(* Logix 5000 AddOnInstructionDefinition export Banner_WLS_Param_v4; software revision 33.00; part 3 of 3 *)
(* tags used below, declared in another part *)
   WLS : Banner_WLS_v4;
   Port_Data : Banner_IOL_Port_v4;
   Port : INT;   // Port Number that device is plugged into.
   Type : SINT;   // 0 = WLS27, 1 = WLS15, 2 = WLF
   Local_Control : DINT;
   Command_Being_Processed : BOOL;
   Update_Archive : BOOL;
   Index_Write_Inprocess : DINT;
   Inprocess_Index : DINT;
   SW_Index : DINT;
   LTW_Index : DINT;
   GW_Index : DINT;
(* Banner_WLS_Param_v4, continued *)

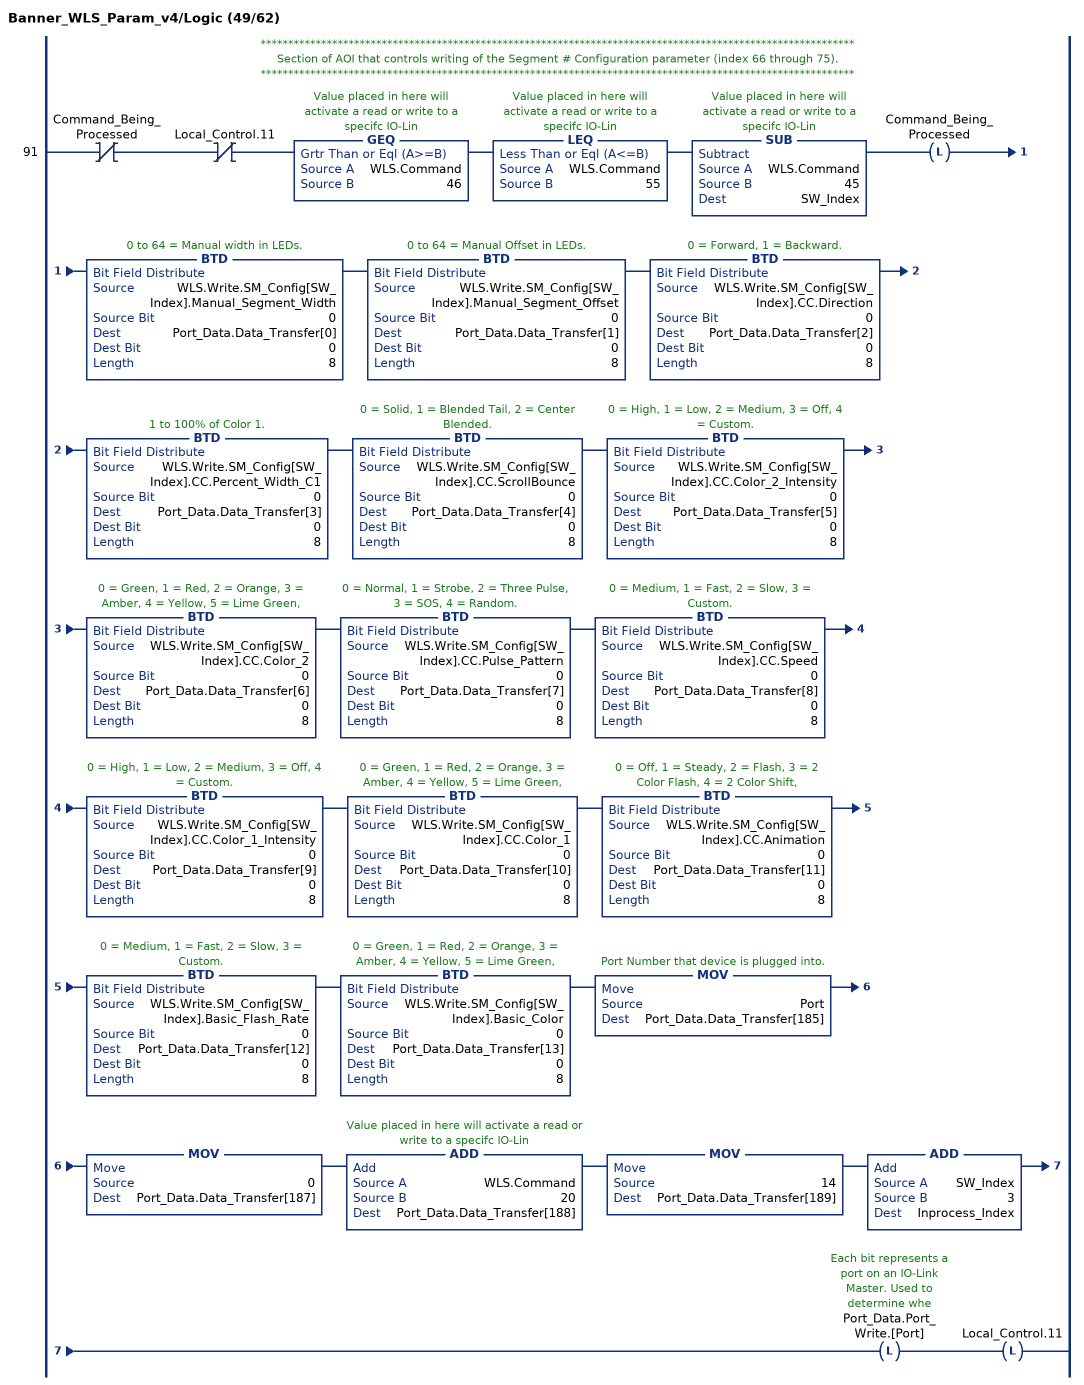
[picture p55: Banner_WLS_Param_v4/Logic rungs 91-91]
   // ************************************************************************************************************
   // Section of AOI that controls writing of the Segment # Configuration parameter (index 66 through 75).
   // ************************************************************************************************************
   91: XIO(Command_Being_Processed)XIO(Local_Control.11)GEQ(WLS.Command,46)LEQ(WLS.Command,55)SUB(WLS.Command,45,SW_Index)OTL(Command_Being_Processed)BTD(WLS.Write.SM_Config[SW_Index].Manual_Segment_Width,0,Port_Data.Data_Transfer[0],0,8)BTD(WLS.Write.SM_Config[SW_Index].Manual_Segment_Offset,0,Port_Data.Data_Transfer[1],0,8)BTD(WLS.Write.SM_Config[SW_Index].CC.Direction,0,Port_Data.Data_Transfer[2],0,8)BTD(WLS.Write.SM_Config[SW_Index].CC.Percent_Width_C1,0,Port_Data.Data_Transfer[3],0,8)BTD(WLS.Write.SM_Config[SW_Index].CC.ScrollBounce,0,Port_Data.Data_Transfer[4],0,8)BTD(WLS.Write.SM_Config[SW_Index].CC.Color_2_Intensity,0,Port_Data.Data_Transfer[5],0,8)BTD(WLS.Write.SM_Config[SW_Index].CC.Color_2,0,Port_Data.Data_Transfer[6],0,8)BTD(WLS.Write.SM_Config[SW_Index].CC.Pulse_Pattern,0,Port_Data.Data_Transfer[7],0,8)BTD(WLS.Write.SM_Config[SW_Index].CC.Speed,0,Port_Data.Data_Transfer[8],0,8)BTD(WLS.Write.SM_Config[SW_Index].CC.Color_1_Intensity,0,Port_Data.Data_Transfer[9],0,8)BTD(WLS.Write.SM_Config[SW_Index].CC.Color_1,0,Port_Data.Data_Transfer[10],0,8)BTD(WLS.Write.SM_Config[SW_Index].CC.Animation,0,Port_Data.Data_Transfer[11],0,8)BTD(WLS.Write.SM_Config[SW_Index].Basic_Flash_Rate,0,Port_Data.Data_Transfer[12],0,8)BTD(WLS.Write.SM_Config[SW_Index].Basic_Color,0,Port_Data.Data_Transfer[13],0,8)MOV(Port,Port_Data.Data_Transfer[185])MOV(0,Port_Data.Data_Transfer[187])ADD(WLS.Command,20,Port_Data.Data_Transfer[188])MOV(14,Port_Data.Data_Transfer[189])ADD(SW_Index,3,Inprocess_Index)OTL(Port_Data.Port_Write.[Port])OTL(Local_Control.11);
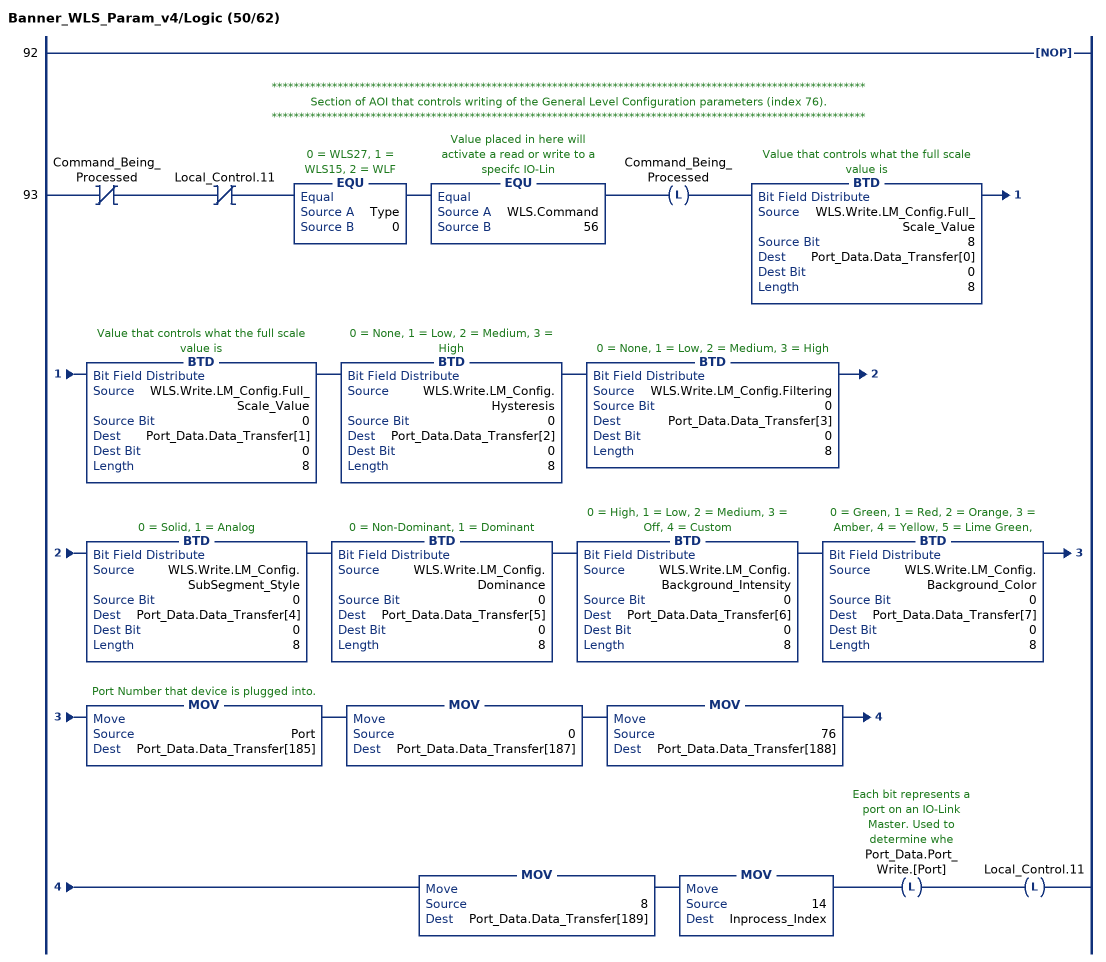
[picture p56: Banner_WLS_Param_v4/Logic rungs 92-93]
   92: NOP();
   // ************************************************************************************************************
   // Section of AOI that controls writing of the General Level Configuration parameters (index 76).
   // ************************************************************************************************************
   93: XIO(Command_Being_Processed)XIO(Local_Control.11)EQU(Type,0)EQU(WLS.Command,56)OTL(Command_Being_Processed)BTD(WLS.Write.LM_Config.Full_Scale_Value,8,Port_Data.Data_Transfer[0],0,8)BTD(WLS.Write.LM_Config.Full_Scale_Value,0,Port_Data.Data_Transfer[1],0,8)BTD(WLS.Write.LM_Config.Hysteresis,0,Port_Data.Data_Transfer[2],0,8)BTD(WLS.Write.LM_Config.Filtering,0,Port_Data.Data_Transfer[3],0,8)BTD(WLS.Write.LM_Config.SubSegment_Style,0,Port_Data.Data_Transfer[4],0,8)BTD(WLS.Write.LM_Config.Dominance,0,Port_Data.Data_Transfer[5],0,8)BTD(WLS.Write.LM_Config.Background_Intensity,0,Port_Data.Data_Transfer[6],0,8)BTD(WLS.Write.LM_Config.Background_Color,0,Port_Data.Data_Transfer[7],0,8)MOV(Port,Port_Data.Data_Transfer[185])MOV(0,Port_Data.Data_Transfer[187])MOV(76,Port_Data.Data_Transfer[188])MOV(8,Port_Data.Data_Transfer[189])MOV(14,Inprocess_Index)OTL(Port_Data.Port_Write.[Port])OTL(Local_Control.11);
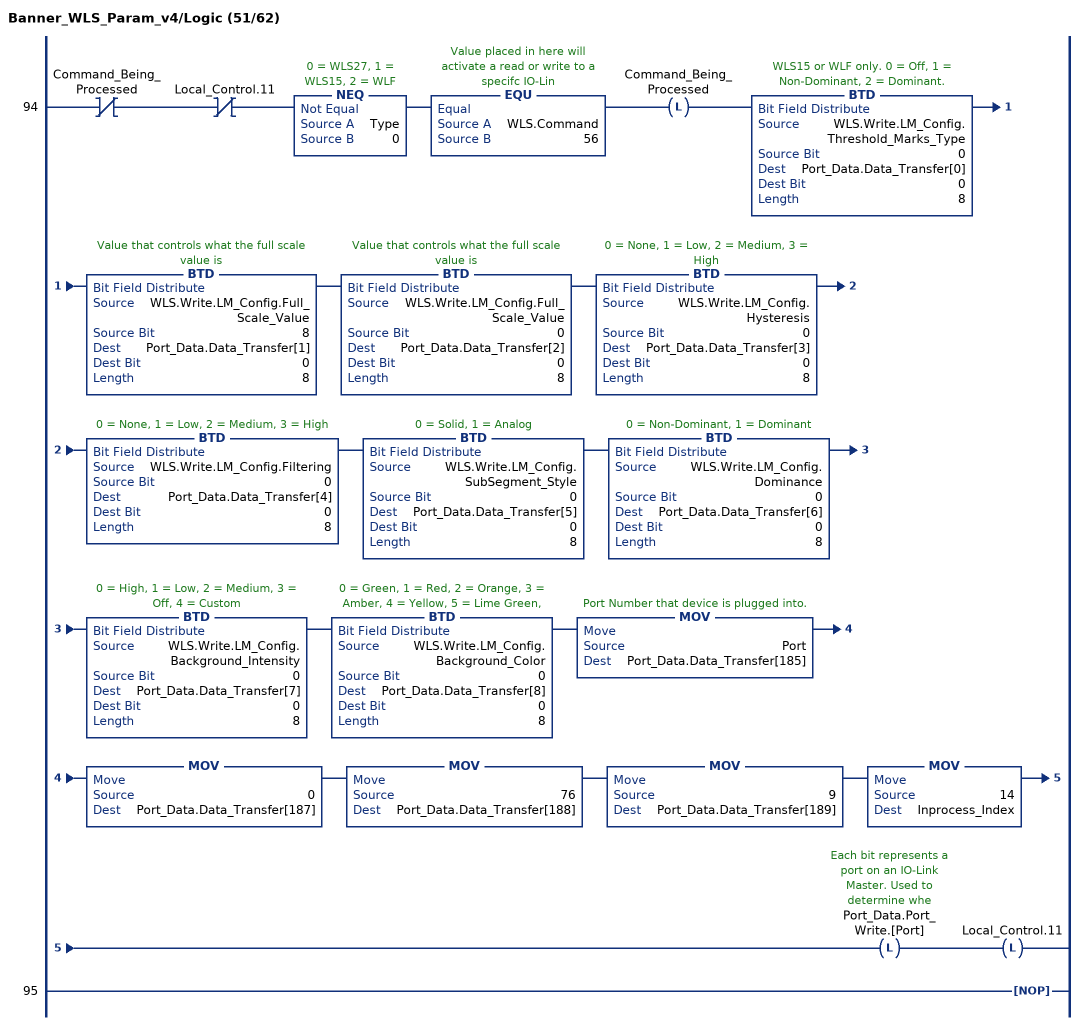
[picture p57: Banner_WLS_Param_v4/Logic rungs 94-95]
   94: XIO(Command_Being_Processed)XIO(Local_Control.11)NEQ(Type,0)EQU(WLS.Command,56)OTL(Command_Being_Processed)BTD(WLS.Write.LM_Config.Threshold_Marks_Type,0,Port_Data.Data_Transfer[0],0,8)BTD(WLS.Write.LM_Config.Full_Scale_Value,8,Port_Data.Data_Transfer[1],0,8)BTD(WLS.Write.LM_Config.Full_Scale_Value,0,Port_Data.Data_Transfer[2],0,8)BTD(WLS.Write.LM_Config.Hysteresis,0,Port_Data.Data_Transfer[3],0,8)BTD(WLS.Write.LM_Config.Filtering,0,Port_Data.Data_Transfer[4],0,8)BTD(WLS.Write.LM_Config.SubSegment_Style,0,Port_Data.Data_Transfer[5],0,8)BTD(WLS.Write.LM_Config.Dominance,0,Port_Data.Data_Transfer[6],0,8)BTD(WLS.Write.LM_Config.Background_Intensity,0,Port_Data.Data_Transfer[7],0,8)BTD(WLS.Write.LM_Config.Background_Color,0,Port_Data.Data_Transfer[8],0,8)MOV(Port,Port_Data.Data_Transfer[185])MOV(0,Port_Data.Data_Transfer[187])MOV(76,Port_Data.Data_Transfer[188])MOV(9,Port_Data.Data_Transfer[189])MOV(14,Inprocess_Index)OTL(Port_Data.Port_Write.[Port])OTL(Local_Control.11);
   95: NOP();
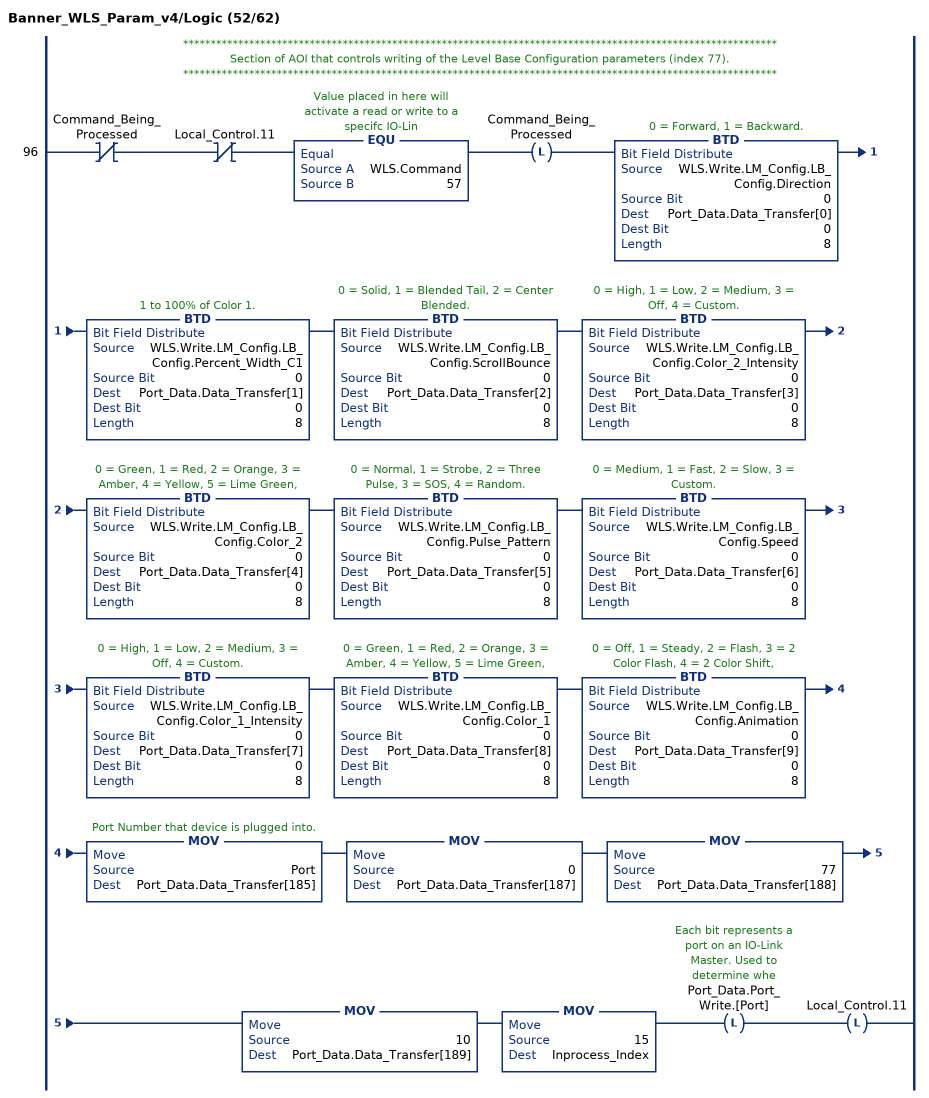
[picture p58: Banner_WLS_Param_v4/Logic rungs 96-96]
   // ************************************************************************************************************
   // Section of AOI that controls writing of the Level Base Configuration parameters (index 77).
   // ************************************************************************************************************
   96: XIO(Command_Being_Processed)XIO(Local_Control.11)EQU(WLS.Command,57)OTL(Command_Being_Processed)BTD(WLS.Write.LM_Config.LB_Config.Direction,0,Port_Data.Data_Transfer[0],0,8)BTD(WLS.Write.LM_Config.LB_Config.Percent_Width_C1,0,Port_Data.Data_Transfer[1],0,8)BTD(WLS.Write.LM_Config.LB_Config.ScrollBounce,0,Port_Data.Data_Transfer[2],0,8)BTD(WLS.Write.LM_Config.LB_Config.Color_2_Intensity,0,Port_Data.Data_Transfer[3],0,8)BTD(WLS.Write.LM_Config.LB_Config.Color_2,0,Port_Data.Data_Transfer[4],0,8)BTD(WLS.Write.LM_Config.LB_Config.Pulse_Pattern,0,Port_Data.Data_Transfer[5],0,8)BTD(WLS.Write.LM_Config.LB_Config.Speed,0,Port_Data.Data_Transfer[6],0,8)BTD(WLS.Write.LM_Config.LB_Config.Color_1_Intensity,0,Port_Data.Data_Transfer[7],0,8)BTD(WLS.Write.LM_Config.LB_Config.Color_1,0,Port_Data.Data_Transfer[8],0,8)BTD(WLS.Write.LM_Config.LB_Config.Animation,0,Port_Data.Data_Transfer[9],0,8)MOV(Port,Port_Data.Data_Transfer[185])MOV(0,Port_Data.Data_Transfer[187])MOV(77,Port_Data.Data_Transfer[188])MOV(10,Port_Data.Data_Transfer[189])MOV(15,Inprocess_Index)OTL(Port_Data.Port_Write.[Port])OTL(Local_Control.11);
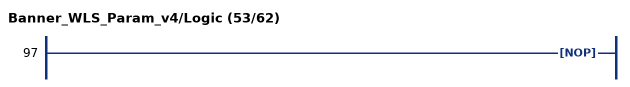
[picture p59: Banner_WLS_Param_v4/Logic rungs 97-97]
   97: NOP();
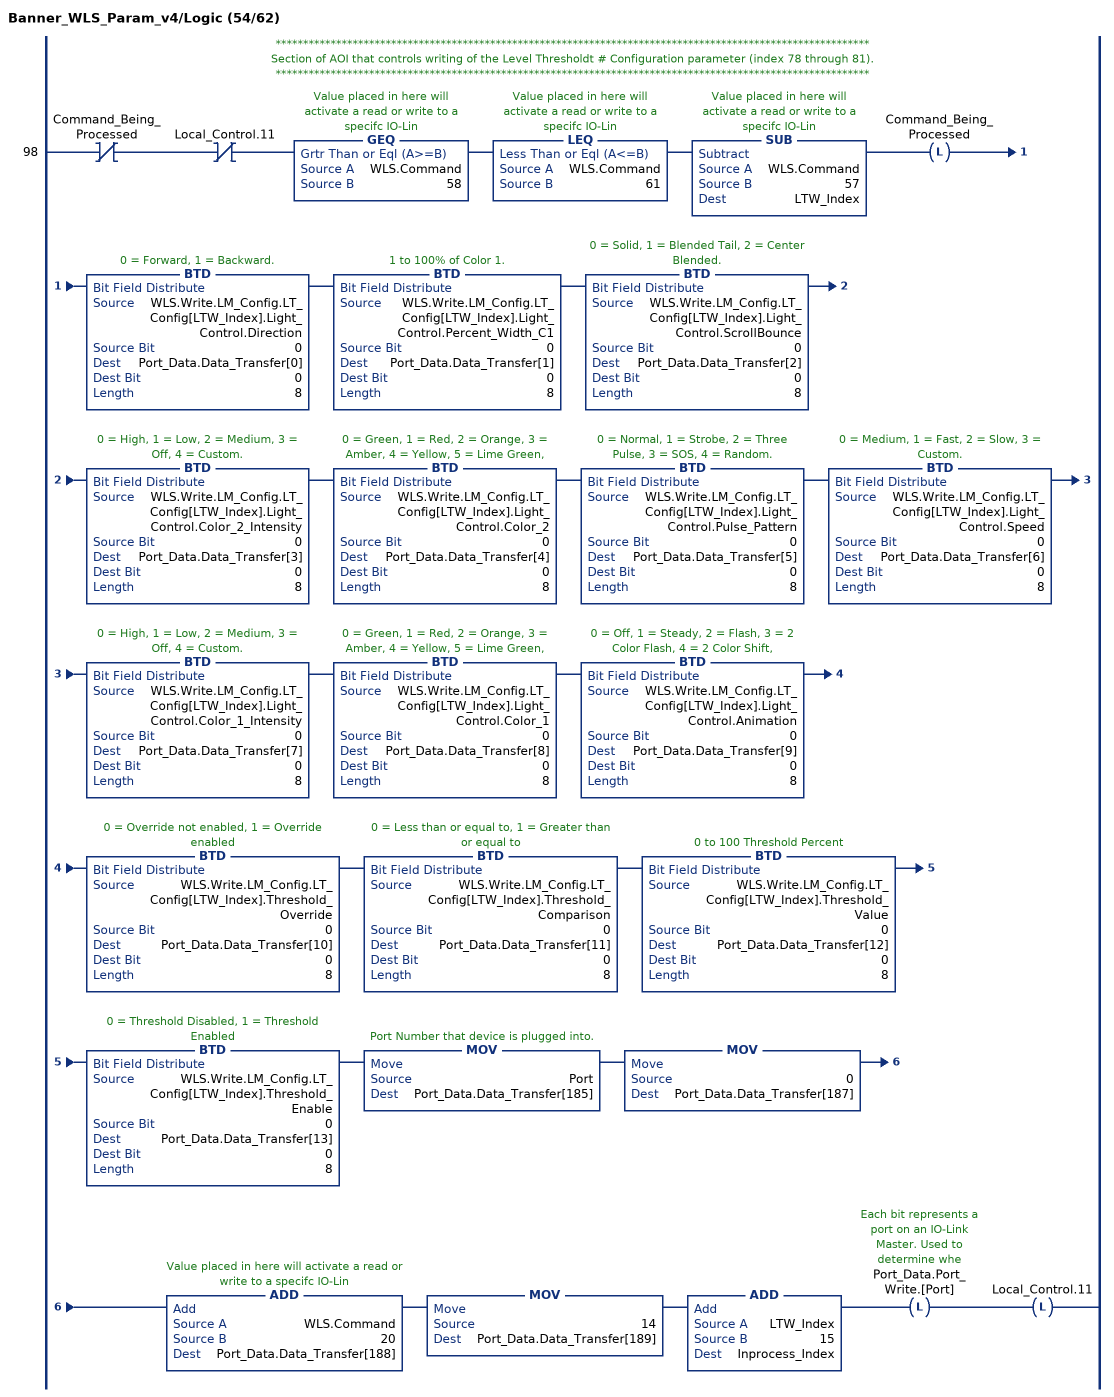
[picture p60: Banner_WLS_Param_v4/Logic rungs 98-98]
   // ************************************************************************************************************
   // Section of AOI that controls writing of the Level Thresholdt # Configuration parameter (index 78 through 81).
   // ************************************************************************************************************
   98: XIO(Command_Being_Processed)XIO(Local_Control.11)GEQ(WLS.Command,58)LEQ(WLS.Command,61)SUB(WLS.Command,57,LTW_Index)OTL(Command_Being_Processed)BTD(WLS.Write.LM_Config.LT_Config[LTW_Index].Light_Control.Direction,0,Port_Data.Data_Transfer[0],0,8)BTD(WLS.Write.LM_Config.LT_Config[LTW_Index].Light_Control.Percent_Width_C1,0,Port_Data.Data_Transfer[1],0,8)BTD(WLS.Write.LM_Config.LT_Config[LTW_Index].Light_Control.ScrollBounce,0,Port_Data.Data_Transfer[2],0,8)BTD(WLS.Write.LM_Config.LT_Config[LTW_Index].Light_Control.Color_2_Intensity,0,Port_Data.Data_Transfer[3],0,8)BTD(WLS.Write.LM_Config.LT_Config[LTW_Index].Light_Control.Color_2,0,Port_Data.Data_Transfer[4],0,8)BTD(WLS.Write.LM_Config.LT_Config[LTW_Index].Light_Control.Pulse_Pattern,0,Port_Data.Data_Transfer[5],0,8)BTD(WLS.Write.LM_Config.LT_Config[LTW_Index].Light_Control.Speed,0,Port_Data.Data_Transfer[6],0,8)BTD(WLS.Write.LM_Config.LT_Config[LTW_Index].Light_Control.Color_1_Intensity,0,Port_Data.Data_Transfer[7],0,8)BTD(WLS.Write.LM_Config.LT_Config[LTW_Index].Light_Control.Color_1,0,Port_Data.Data_Transfer[8],0,8)BTD(WLS.Write.LM_Config.LT_Config[LTW_Index].Light_Control.Animation,0,Port_Data.Data_Transfer[9],0,8)BTD(WLS.Write.LM_Config.LT_Config[LTW_Index].Threshold_Override,0,Port_Data.Data_Transfer[10],0,8)BTD(WLS.Write.LM_Config.LT_Config[LTW_Index].Threshold_Comparison,0,Port_Data.Data_Transfer[11],0,8)BTD(WLS.Write.LM_Config.LT_Config[LTW_Index].Threshold_Value,0,Port_Data.Data_Transfer[12],0,8)BTD(WLS.Write.LM_Config.LT_Config[LTW_Index].Threshold_Enable,0,Port_Data.Data_Transfer[13],0,8)MOV(Port,Port_Data.Data_Transfer[185])MOV(0,Port_Data.Data_Transfer[187])ADD(WLS.Command,20,Port_Data.Data_Transfer[188])MOV(14,Port_Data.Data_Transfer[189])ADD(LTW_Index,15,Inprocess_Index)OTL(Port_Data.Port_Write.[Port])OTL(Local_Control.11);
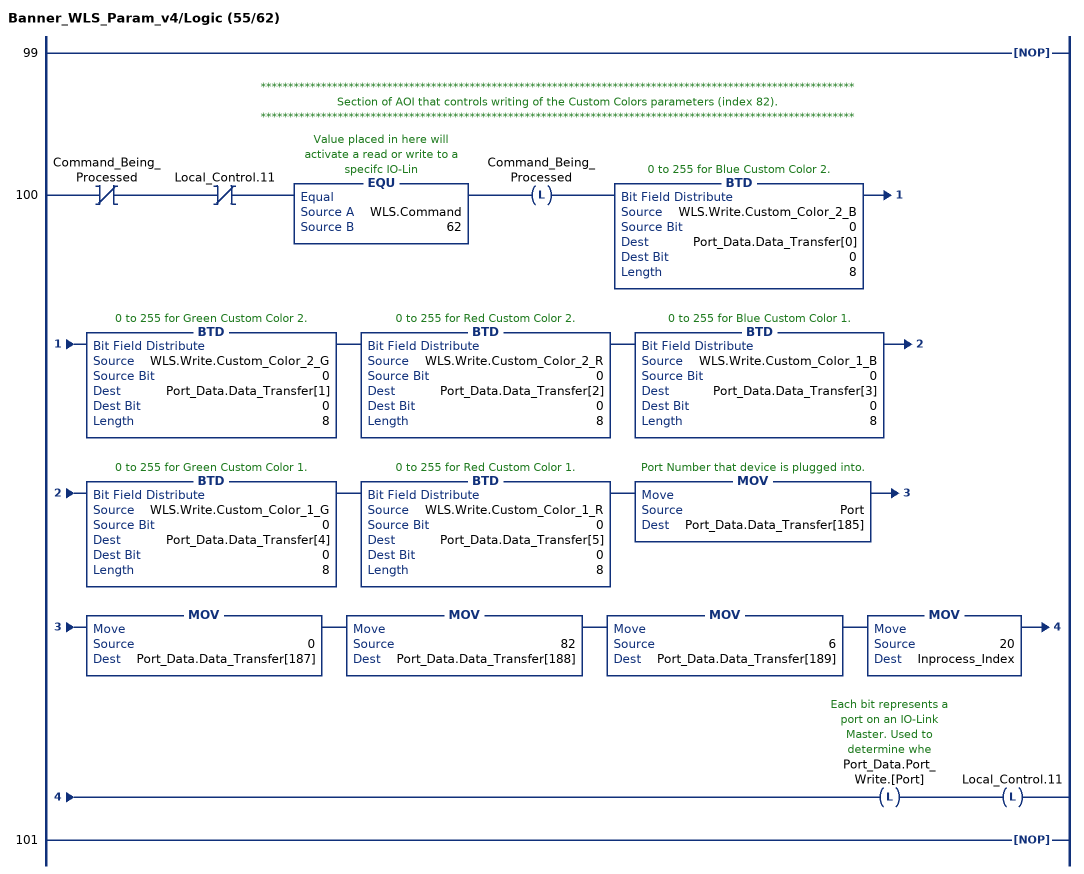
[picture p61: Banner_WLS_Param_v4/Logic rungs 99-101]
   99: NOP();
   // ************************************************************************************************************
   // Section of AOI that controls writing of the Custom Colors parameters (index 82).
   // ************************************************************************************************************
   100: XIO(Command_Being_Processed)XIO(Local_Control.11)EQU(WLS.Command,62)OTL(Command_Being_Processed)BTD(WLS.Write.Custom_Color_2_B,0,Port_Data.Data_Transfer[0],0,8)BTD(WLS.Write.Custom_Color_2_G,0,Port_Data.Data_Transfer[1],0,8)BTD(WLS.Write.Custom_Color_2_R,0,Port_Data.Data_Transfer[2],0,8)BTD(WLS.Write.Custom_Color_1_B,0,Port_Data.Data_Transfer[3],0,8)BTD(WLS.Write.Custom_Color_1_G,0,Port_Data.Data_Transfer[4],0,8)BTD(WLS.Write.Custom_Color_1_R,0,Port_Data.Data_Transfer[5],0,8)MOV(Port,Port_Data.Data_Transfer[185])MOV(0,Port_Data.Data_Transfer[187])MOV(82,Port_Data.Data_Transfer[188])MOV(6,Port_Data.Data_Transfer[189])MOV(20,Inprocess_Index)OTL(Port_Data.Port_Write.[Port])OTL(Local_Control.11);
   101: NOP();
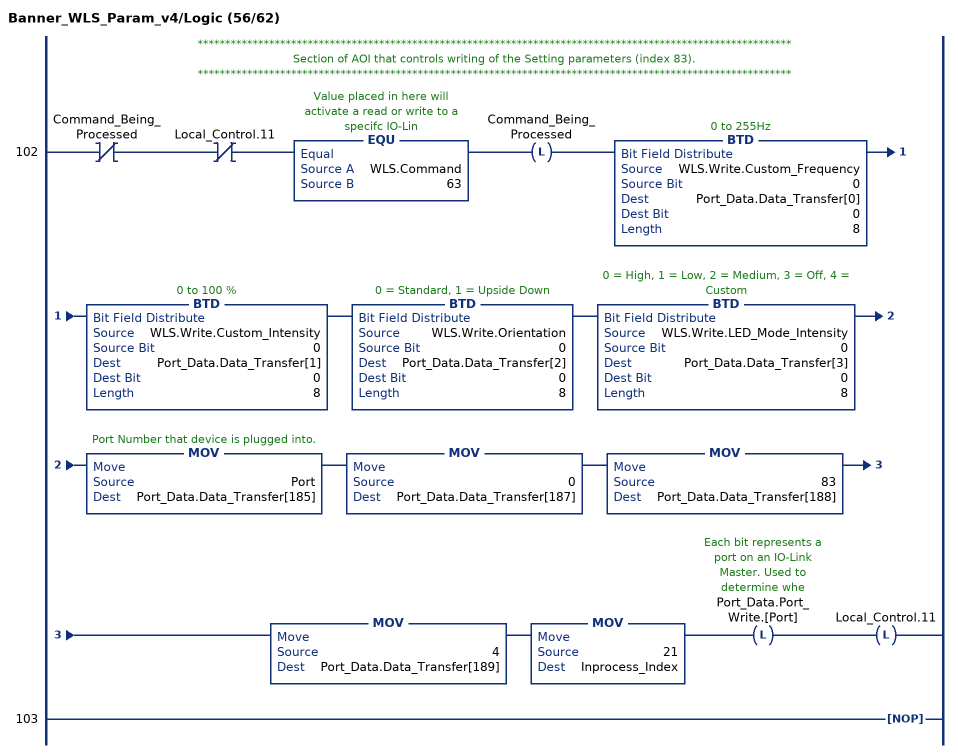
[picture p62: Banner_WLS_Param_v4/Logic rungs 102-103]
   // ************************************************************************************************************
   // Section of AOI that controls writing of the Setting parameters (index 83).
   // ************************************************************************************************************
   102: XIO(Command_Being_Processed)XIO(Local_Control.11)EQU(WLS.Command,63)OTL(Command_Being_Processed)BTD(WLS.Write.Custom_Frequency,0,Port_Data.Data_Transfer[0],0,8)BTD(WLS.Write.Custom_Intensity,0,Port_Data.Data_Transfer[1],0,8)BTD(WLS.Write.Orientation,0,Port_Data.Data_Transfer[2],0,8)BTD(WLS.Write.LED_Mode_Intensity,0,Port_Data.Data_Transfer[3],0,8)MOV(Port,Port_Data.Data_Transfer[185])MOV(0,Port_Data.Data_Transfer[187])MOV(83,Port_Data.Data_Transfer[188])MOV(4,Port_Data.Data_Transfer[189])MOV(21,Inprocess_Index)OTL(Port_Data.Port_Write.[Port])OTL(Local_Control.11);
   103: NOP();
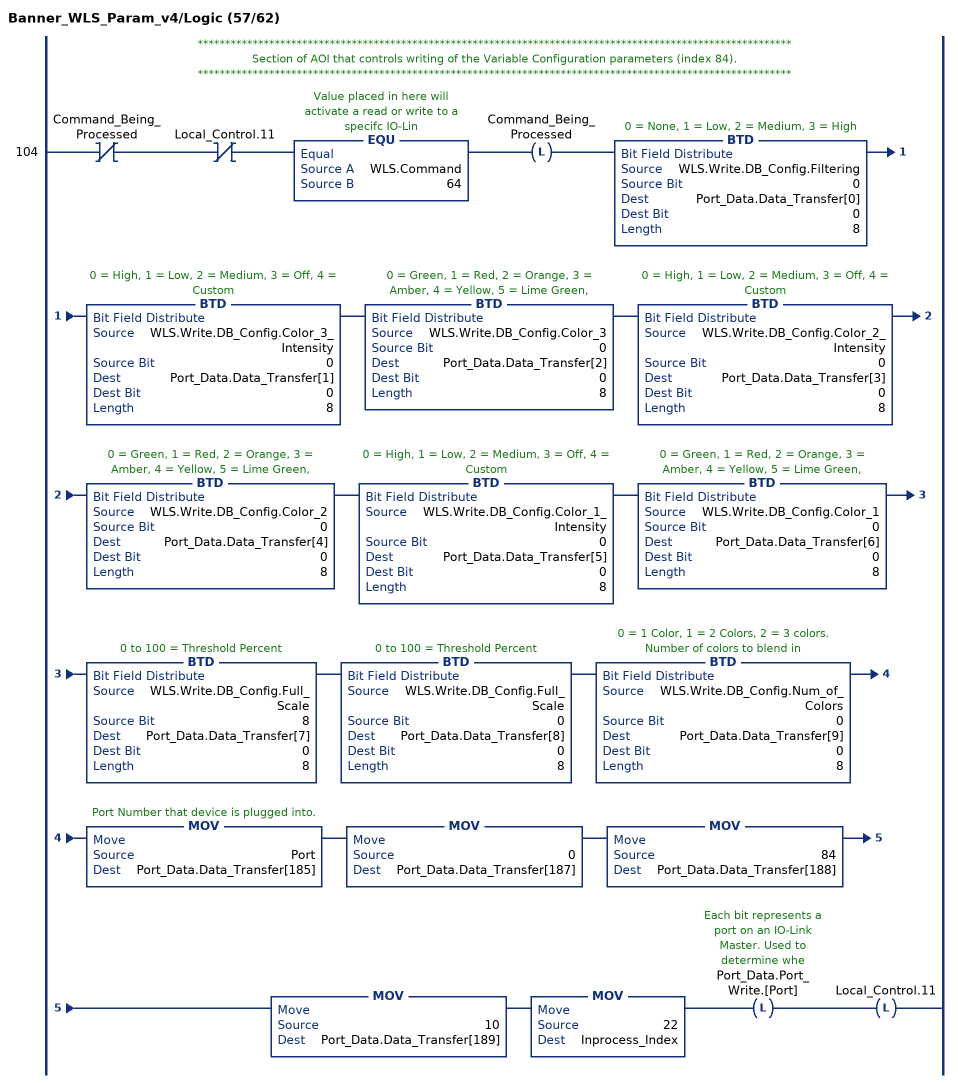
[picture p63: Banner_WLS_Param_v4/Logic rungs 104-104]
   // ************************************************************************************************************
   // Section of AOI that controls writing of the Variable Configuration parameters (index 84).
   // ************************************************************************************************************
   104: XIO(Command_Being_Processed)XIO(Local_Control.11)EQU(WLS.Command,64)OTL(Command_Being_Processed)BTD(WLS.Write.DB_Config.Filtering,0,Port_Data.Data_Transfer[0],0,8)BTD(WLS.Write.DB_Config.Color_3_Intensity,0,Port_Data.Data_Transfer[1],0,8)BTD(WLS.Write.DB_Config.Color_3,0,Port_Data.Data_Transfer[2],0,8)BTD(WLS.Write.DB_Config.Color_2_Intensity,0,Port_Data.Data_Transfer[3],0,8)BTD(WLS.Write.DB_Config.Color_2,0,Port_Data.Data_Transfer[4],0,8)BTD(WLS.Write.DB_Config.Color_1_Intensity,0,Port_Data.Data_Transfer[5],0,8)BTD(WLS.Write.DB_Config.Color_1,0,Port_Data.Data_Transfer[6],0,8)BTD(WLS.Write.DB_Config.Full_Scale,8,Port_Data.Data_Transfer[7],0,8)BTD(WLS.Write.DB_Config.Full_Scale,0,Port_Data.Data_Transfer[8],0,8)BTD(WLS.Write.DB_Config.Num_of_Colors,0,Port_Data.Data_Transfer[9],0,8)MOV(Port,Port_Data.Data_Transfer[185])MOV(0,Port_Data.Data_Transfer[187])MOV(84,Port_Data.Data_Transfer[188])MOV(10,Port_Data.Data_Transfer[189])MOV(22,Inprocess_Index)OTL(Port_Data.Port_Write.[Port])OTL(Local_Control.11);
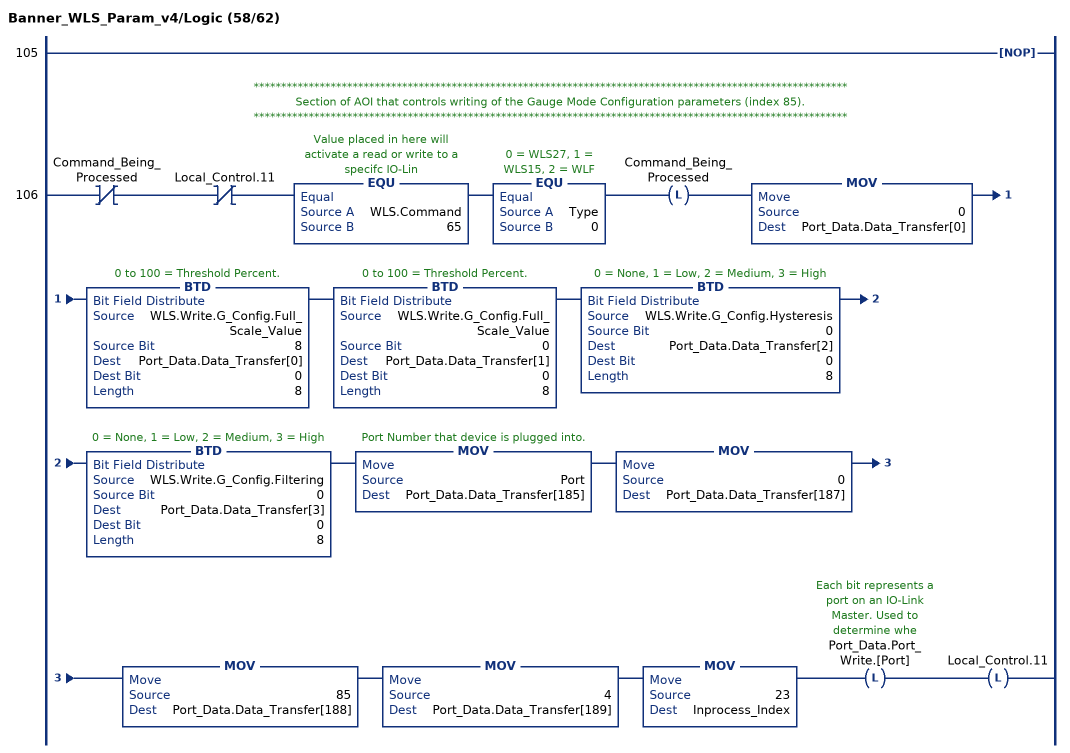
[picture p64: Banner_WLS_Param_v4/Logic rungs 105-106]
   105: NOP();
   // ************************************************************************************************************
   // Section of AOI that controls writing of the Gauge Mode Configuration parameters (index 85).
   // ************************************************************************************************************
   106: XIO(Command_Being_Processed)XIO(Local_Control.11)EQU(WLS.Command,65)EQU(Type,0)OTL(Command_Being_Processed)MOV(0,Port_Data.Data_Transfer[0])BTD(WLS.Write.G_Config.Full_Scale_Value,8,Port_Data.Data_Transfer[0],0,8)BTD(WLS.Write.G_Config.Full_Scale_Value,0,Port_Data.Data_Transfer[1],0,8)BTD(WLS.Write.G_Config.Hysteresis,0,Port_Data.Data_Transfer[2],0,8)BTD(WLS.Write.G_Config.Filtering,0,Port_Data.Data_Transfer[3],0,8)MOV(Port,Port_Data.Data_Transfer[185])MOV(0,Port_Data.Data_Transfer[187])MOV(85,Port_Data.Data_Transfer[188])MOV(4,Port_Data.Data_Transfer[189])MOV(23,Inprocess_Index)OTL(Port_Data.Port_Write.[Port])OTL(Local_Control.11);
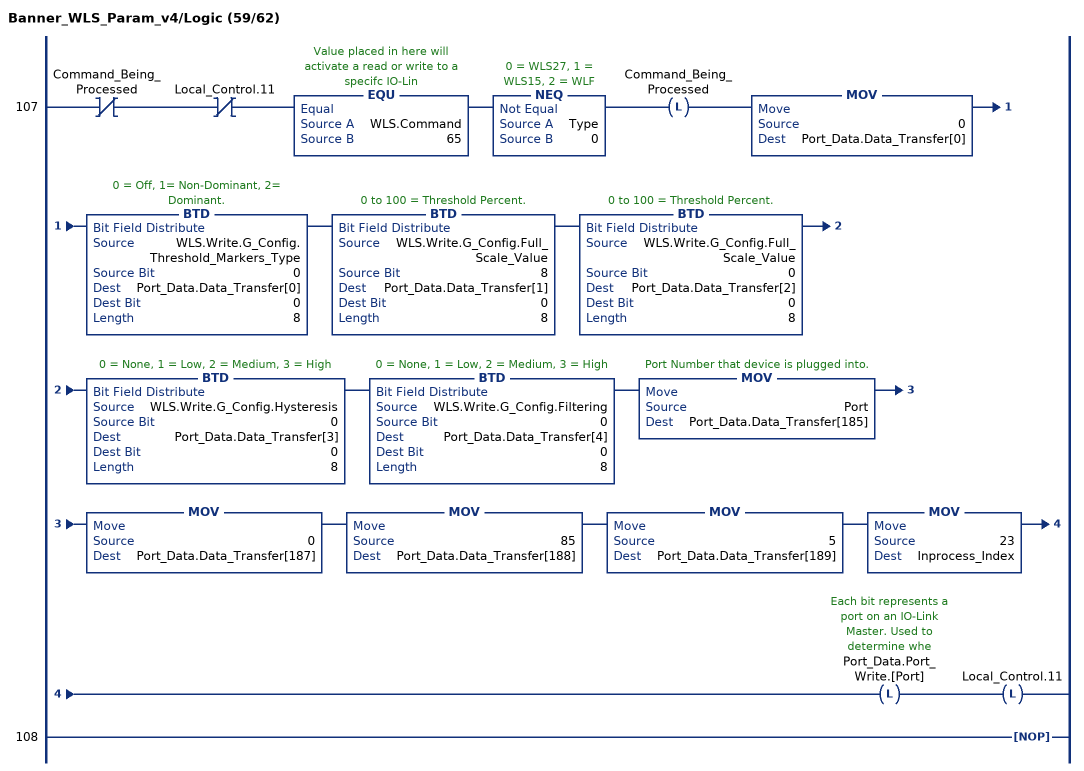
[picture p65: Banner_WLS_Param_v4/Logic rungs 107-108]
   107: XIO(Command_Being_Processed)XIO(Local_Control.11)EQU(WLS.Command,65)NEQ(Type,0)OTL(Command_Being_Processed)MOV(0,Port_Data.Data_Transfer[0])BTD(WLS.Write.G_Config.Threshold_Markers_Type,0,Port_Data.Data_Transfer[0],0,8)BTD(WLS.Write.G_Config.Full_Scale_Value,8,Port_Data.Data_Transfer[1],0,8)BTD(WLS.Write.G_Config.Full_Scale_Value,0,Port_Data.Data_Transfer[2],0,8)BTD(WLS.Write.G_Config.Hysteresis,0,Port_Data.Data_Transfer[3],0,8)BTD(WLS.Write.G_Config.Filtering,0,Port_Data.Data_Transfer[4],0,8)MOV(Port,Port_Data.Data_Transfer[185])MOV(0,Port_Data.Data_Transfer[187])MOV(85,Port_Data.Data_Transfer[188])MOV(5,Port_Data.Data_Transfer[189])MOV(23,Inprocess_Index)OTL(Port_Data.Port_Write.[Port])OTL(Local_Control.11);
   108: NOP();
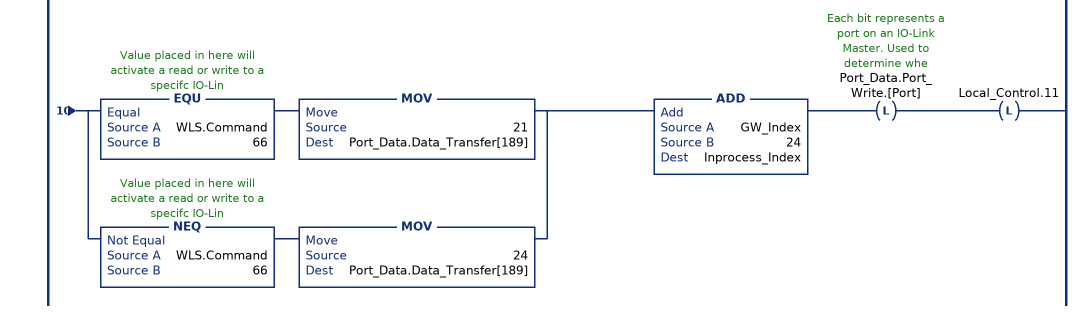
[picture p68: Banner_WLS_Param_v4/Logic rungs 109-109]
   // *****************************************************************************************************************************************************************************
   // Section of AOI that controls writing of the Gauge Mode Center Settings parameters (index 86), Gauge Mode Threshold 1 & 2 Settings (Index 87 &88).
   // *****************************************************************************************************************************************************************************
   109: XIO(Command_Being_Processed)XIO(Local_Control.11)GEQ(WLS.Command,66)LEQ(WLS.Command,68)SUB(WLS.Command,66,GW_Index)OTL(Command_Being_Processed)BTD(WLS.Write.G_Config.CC[GW_Index].Back_CC.Direction,0,Port_Data.Data_Transfer[0],0,8)BTD(WLS.Write.G_Config.CC[GW_Index].Back_CC.Percent_Width_C1,0,Port_Data.Data_Transfer[1],0,8)BTD(WLS.Write.G_Config.CC[GW_Index].Back_CC.ScrollBounce,0,Port_Data.Data_Transfer[2],0,8)BTD(WLS.Write.G_Config.CC[GW_Index].Back_CC.Color_2_Intensity,0,Port_Data.Data_Transfer[3],0,8)BTD(WLS.Write.G_Config.CC[GW_Index].Back_CC.Color_2,0,Port_Data.Data_Transfer[4],0,8)BTD(WLS.Write.G_Config.CC[GW_Index].Back_CC.Pulse_Pattern,0,Port_Data.Data_Transfer[5],0,8)BTD(WLS.Write.G_Config.CC[GW_Index].Back_CC.Speed,0,Port_Data.Data_Transfer[6],0,8)BTD(WLS.Write.G_Config.CC[GW_Index].Back_CC.Color_1_Intensity,0,Port_Data.Data_Transfer[7],0,8)BTD(WLS.Write.G_Config.CC[GW_Index].Back_CC.Color_1,0,Port_Data.Data_Transfer[8],0,8)BTD(WLS.Write.G_Config.CC[GW_Index].Back_CC.Animation,0,Port_Data.Data_Transfer[9],0,8)BTD(WLS.Write.G_Config.CC[GW_Index].Main_CC.Direction,0,Port_Data.Data_Transfer[10],0,8)BTD(WLS.Write.G_Config.CC[GW_Index].Main_CC.Percent_Width_C1,0,Port_Data.Data_Transfer[11],0,8)BTD(WLS.Write.G_Config.CC[GW_Index].Main_CC.ScrollBounce,0,Port_Data.Data_Transfer[12],0,8)BTD(WLS.Write.G_Config.CC[GW_Index].Main_CC.Color_2_Intensity,0,Port_Data.Data_Transfer[13],0,8)BTD(WLS.Write.G_Config.CC[GW_Index].Main_CC.Color_2,0,Port_Data.Data_Transfer[14],0,8)BTD(WLS.Write.G_Config.CC[GW_Index].Main_CC.Pulse_Pattern,0,Port_Data.Data_Transfer[15],0,8)BTD(WLS.Write.G_Config.CC[GW_Index].Main_CC.Speed,0,Port_Data.Data_Transfer[16],0,8)BTD(WLS.Write.G_Config.CC[GW_Index].Main_CC.Color_1_Intensity,0,Port_Data.Data_Transfer[17],0,8)BTD(WLS.Write.G_Config.CC[GW_Index].Main_CC.Color_1,0,Port_Data.Data_Transfer[18],0,8)BTD(WLS.Write.G_Config.CC[GW_Index].Main_CC.Animation,0,Port_Data.Data_Transfer[19],0,8)BTD(WLS.Write.G_Config.CC[GW_Index].Percent_Width_of_Main_Segment,0,Port_Data.Data_Transfer[20],0,8)BTD(WLS.Write.G_Config.CC[GW_Index].Threshold_Comparison,0,Port_Data.Data_Transfer[21],0,8)BTD(WLS.Write.G_Config.CC[GW_Index].Threshold_Value_Percent,0,Port_Data.Data_Transfer[22],0,8)BTD(WLS.Write.G_Config.CC[GW_Index].Threshold_Enable,0,Port_Data.Data_Transfer[23],0,8)MOV(Port,Port_Data.Data_Transfer[185])MOV(0,Port_Data.Data_Transfer[187])ADD(WLS.Command,20,Port_Data.Data_Transfer[188])[EQU(WLS.Command,66) MOV(21,Port_Data.Data_Transfer[189]) ,NEQ(WLS.Command,66) MOV(24,Port_Data.Data_Transfer[189]) ]ADD(GW_Index,24,Inprocess_Index)OTL(Port_Data.Port_Write.[Port])OTL(Local_Control.11);
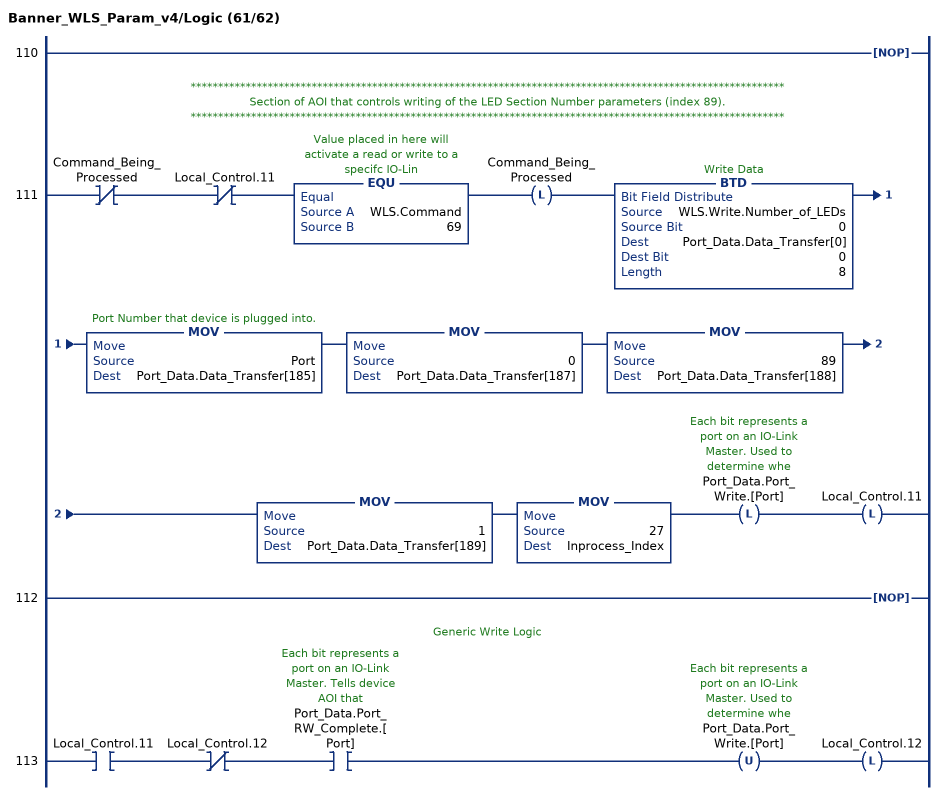
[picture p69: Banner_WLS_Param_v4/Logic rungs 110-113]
   110: NOP();
   // ************************************************************************************************************
   // Section of AOI that controls writing of the LED Section Number parameters (index 89).
   // ************************************************************************************************************
   111: XIO(Command_Being_Processed)XIO(Local_Control.11)EQU(WLS.Command,69)OTL(Command_Being_Processed)BTD(WLS.Write.Number_of_LEDs,0,Port_Data.Data_Transfer[0],0,8)MOV(Port,Port_Data.Data_Transfer[185])MOV(0,Port_Data.Data_Transfer[187])MOV(89,Port_Data.Data_Transfer[188])MOV(1,Port_Data.Data_Transfer[189])MOV(27,Inprocess_Index)OTL(Port_Data.Port_Write.[Port])OTL(Local_Control.11);
   112: NOP();
   // Generic Write Logic
   113: XIC(Local_Control.11)XIO(Local_Control.12)XIC(Port_Data.Port_RW_Complete.[Port])OTU(Port_Data.Port_Write.[Port])OTL(Local_Control.12);
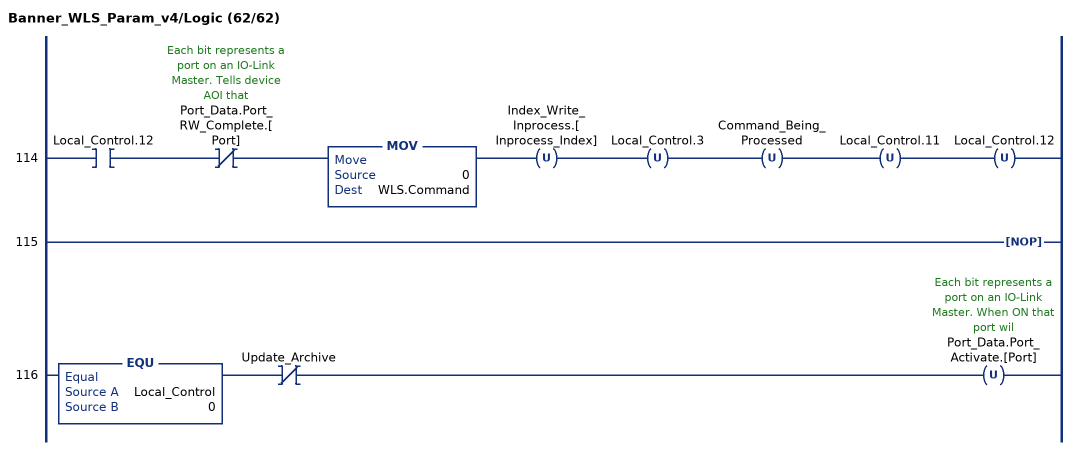
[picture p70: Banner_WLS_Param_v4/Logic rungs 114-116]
   114: XIC(Local_Control.12)XIO(Port_Data.Port_RW_Complete.[Port])MOV(0,WLS.Command)OTU(Index_Write_Inprocess.[Inprocess_Index])OTU(Local_Control.3)OTU(Command_Being_Processed)OTU(Local_Control.11)OTU(Local_Control.12);
   115: NOP();
   116: EQU(Local_Control,0)XIO(Update_Archive)OTU(Port_Data.Port_Activate.[Port]);
END_ROUTINE
END_ADD_ON_INSTRUCTION
